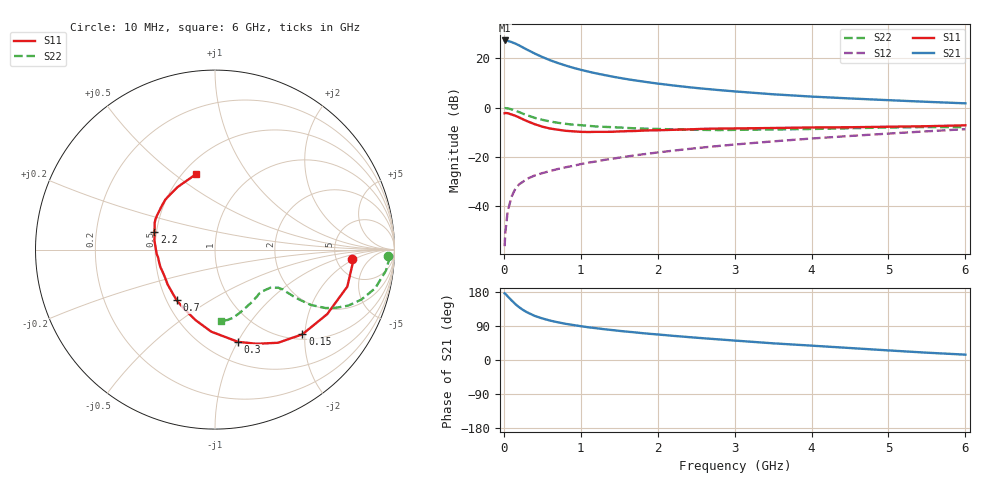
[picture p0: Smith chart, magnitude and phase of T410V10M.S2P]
! Infineon Technologies  Discrete & RF Semiconductors
! BFR182T
! Si NPN RF Bipolar Junction Transistor in SC75
! VCE = 10 V  IC = 10 mA
! Common Emitter S-Parameters:  October  1999
# GHz  S  MA  R  50
!  f  S11  S21  S12  S22
! GHz  MAG  ANG  MAG  ANG  MAG  ANG  MAG  ANG
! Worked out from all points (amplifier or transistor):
!   36 points, 10 MHz to 6 GHz, reference 50 ohm
!   highest |S21| = 27.3 dB at 10 MHz (marker M1)
!   |S21| within 3 dB of that: start of sweep to 257 MHz
!   unconditionally stable (mu >= 1): 1.134 GHz to 4.059 GHz
!   at 250 MHz: K = 0.42, MSG = 27.3 dB, |S12| = -30.2 dB
!   at 1.4 GHz: K = 1.05, MAG = 15.5 dB, |S12| = -20.9 dB
!   at 6 GHz: K = 0.87, MSG = 5.3 dB, |S12| = -8.8 dB
!   S11 on the Smith chart (normalised r, x): 10 MHz: 7.00, -1.84; 150 MHz: 1.11, -1.94; 300 MHz: 0.70, -1.01; 700 MHz: 0.56, -0.36; 2.2 GHz: 0.49, +0.11; 6 GHz: 0.58, +0.60
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0.01  0.7646 -4.1  23.2 175.9  0.0015 79.2  0.9667 -2.2
0.02  0.7724 -4.9  22.96 174.8  0.0029 80.3  0.973 -2.9
0.05  0.7656 -15.6  22.73 167.9  0.0077 82.9  0.9591 -7.1
0.1  0.7211 -29.9  21.51 157.4  0.0152 74.8  0.9179 -13.6
0.15  0.6782 -44.1  20.02 147.4  0.0222 70.7  0.8611 -18.9
0.2  0.6268 -55.9  18.35 139.1  0.0274 68.0  0.8055 -22.8
0.25  0.5739 -66.1  16.65 132.1  0.0309 62.5  0.7472 -25.7
0.3  0.5301 -75.9  15.13 126.1  0.0352 61.2  0.6985 -27.8
0.4  0.4578 -92.6  12.6 116.5  0.0412 58.8  0.6169 -30.0
0.5  0.4074 -105.5  10.68 109.7  0.0461 58.5  0.5617 -30.5
0.6  0.3734 -117.1  9.196 104.1  0.0508 58.5  0.5201 -30.9
0.7  0.3539 -127.2  8.082 99.6  0.0559 59.8  0.4893 -30.7
0.9  0.3273 -144.0  6.45 92.4  0.0647 61.3  0.4472 -30.6
1.1  0.3169 -157.6  5.377 86.3  0.0753 62.2  0.4234 -30.9
1.3  0.3194 -168.2  4.609 81.4  0.0854 63.5  0.4038 -31.7
1.6  0.3296 179.7  3.784 74.9  0.1006 64.0  0.3835 -33.2
2.2  0.3516 163.8  2.814 63.8  0.1322 64.6  0.3597 -38.7
2.8  0.3724 152.8  2.262 54.3  0.1651 63.6  0.3472 -45.5
3.5  0.3824 141.6  1.86 44.0  0.2043 61.5  0.3569 -54.4
4.5  0.3963 128.5  1.529 31.6  0.2633 57.3  0.3776 -68.3
5.5  0.416 111.8  1.306 19.3  0.3277 52.4  0.3983 -80.1
6  0.4336 104.0  1.216 14.1  0.3618 49.1  0.3994 -84.8
